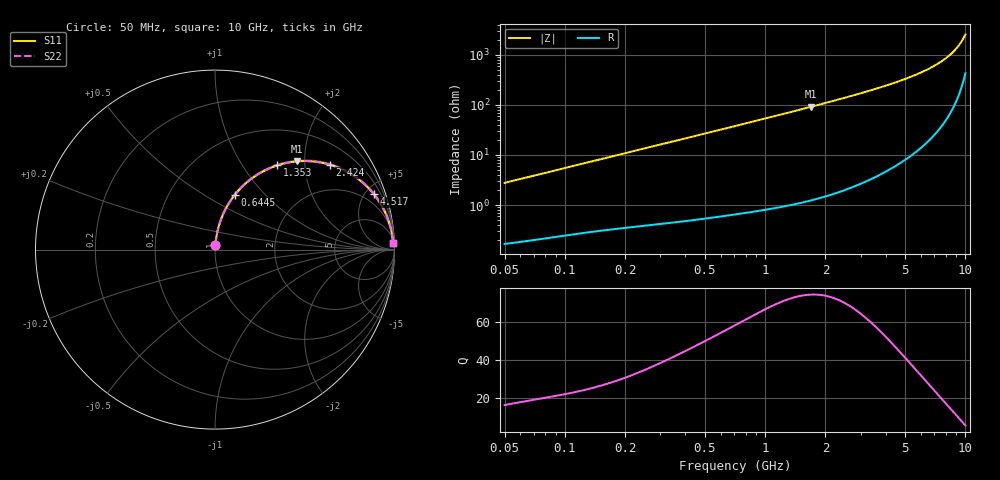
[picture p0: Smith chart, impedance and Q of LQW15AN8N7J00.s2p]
!Murata Part Number: LQW15AN8N7J00
!These Parameters are Measured in Series Mode Connection
!  o--[Z]--o
!Port1  Port2
!  o-------o
!Freq. Start=50[MHz] Stop=10[GHz], 401[Steps]
# Hz S RI R 50
!Freq.(Hz)	S 11(Real)	S 11(Imag)	S 21(Real)	S 21(Imag)	S 12(Real)	S 12(Imag)	S 22(Real)	S 22(Imag)
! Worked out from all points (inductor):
!   401 points, 50 MHz to 10 GHz, reference 50 ohm
!   read as one part in series: L = 8.76 nH near 51.34 MHz
!   highest Q = 74.2 at 1.695 GHz (marker M1), where L = 8.61 nH
!   S11 on the Smith chart (normalised r, x): 50 MHz: 1.00, +0.06; 644.5 MHz: 1.01, +0.69; 1.353 GHz: 1.02, +1.45; 2.424 GHz: 1.04, +2.69; 4.517 GHz: 1.12, +5.69; 10 GHz: 10, +50
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5e7  0.00243 0.0275  0.9976 -0.0275  0.9976 -0.0275  0.00243 0.0275
1.214486e8  0.00703 0.0653  0.993 -0.0653  0.993 -0.0653  0.00703 0.0653
1.930779e8  0.014 0.1022  0.986 -0.1022  0.986 -0.1022  0.014 0.1022
2.949953e8  0.0282 0.1529  0.9718 -0.1529  0.9718 -0.1529  0.0282 0.1529
4.507103e8  0.0589 0.2252  0.9411 -0.2252  0.9411 -0.2252  0.0589 0.2252
6.444912e8  0.1099 0.3039  0.8901 -0.3039  0.8901 -0.3039  0.1099 0.3039
7.071068e8  0.1286 0.3263  0.8714 -0.3263  0.8714 -0.3263  0.1286 0.3263
9.846897e8  0.2201 0.4068  0.7799 -0.4068  0.7799 -0.4068  0.2201 0.4068
1.353197e9  0.3475 0.4693  0.6525 -0.4693  0.6525 -0.4693  0.3475 0.4693
1.694942e9  0.4574 0.4915  0.5426 -0.4915  0.5426 -0.4915  0.4574 0.4915
1.717543e9  0.4642 0.492  0.5358 -0.492  0.5358 -0.492  0.4642 0.492
2.423676e9  0.6415 0.4725  0.3585 -0.4725  0.3585 -0.4725  0.6415 0.4725
3.200947e9  0.7685 0.4138  0.2315 -0.4138  0.2315 -0.4138  0.7685 0.4138
4.171863e9  0.8624 0.3346  0.1376 -0.3346  0.1376 -0.3346  0.8624 0.3346
4.516952e9  0.885 0.3084  0.115 -0.3084  0.115 -0.3084  0.885 0.3084
6.045081e9  0.9469 0.2089  0.0531 -0.2089  0.0531 -0.2089  0.9469 0.2089
6.810442e9  0.9639 0.1679  0.0361 -0.1679  0.0361 -0.1679  0.9639 0.1679
7.571744e9  0.9755 0.1317  0.0245 -0.1317  0.0245 -0.1317  0.9755 0.1317
8.307378e9  0.9831 0.1003  0.0169 -0.1003  0.0169 -0.1003  0.9831 0.1003
8.876195e9  0.9872 0.078  0.0128 -0.078  0.0128 -0.078  0.9872 0.078
9.359165e9  0.9898 0.0602  0.0102 -0.0602  0.0102 -0.0602  0.9898 0.0602
1e10  0.992 0.0381  0.008 -0.0381  0.008 -0.0381  0.992 0.0381
